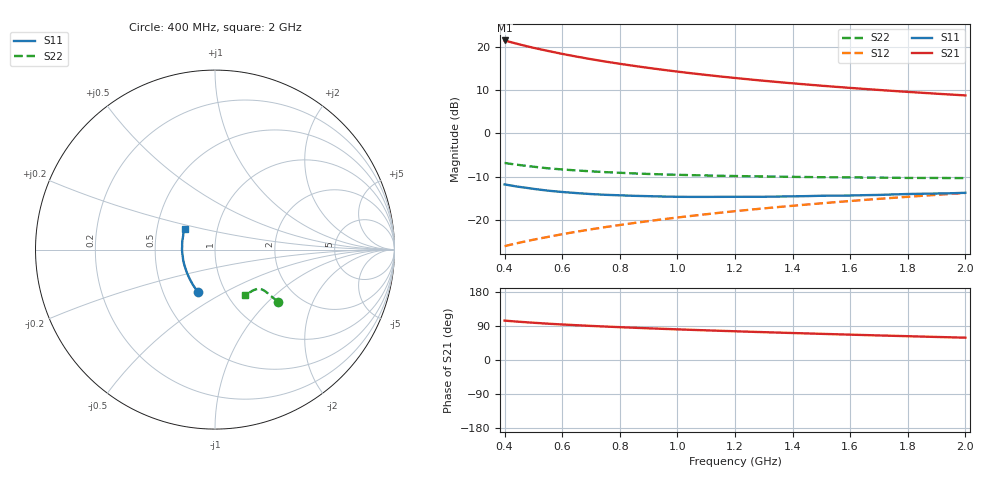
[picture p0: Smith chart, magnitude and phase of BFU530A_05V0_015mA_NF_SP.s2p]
! Filename:  P:\Prog\Test\Noise\ATS_data\Testdata_Net\06 Compressed Noise after Statistics\BFU530A_APG2013_33_A05_05p0V_015mA_NF_CM01_D.sf
! Date/Time: Tue 16/Apr/2013 15:10:56
! BFU530A_APG2013_33_A05_05p0V_1to25mA_NF_CM01_Bias6_R.sf
! Noise Parameter Data File
! BFU530A_APG2013_33_A05_05p0V_1to25mA_NF_CM01
! Date/time: Fri Apr 12 15:27:54 2013
! VAR V_out= 5.001000
! VAR I_out= 15.000000
! VAR V_in= 0.836900
! VAR I_in= 0.162200
! Device data file deembeded for feedlines and parallel
! Original file: \06 Compressed Noise after Statistics\BFU530A_APG2013_33_A05_05p0V_015mA_NF_CM01_R.sf
! Feed-files: PR017V01_150413_Feed1.s2p, PR017V01_150413_Feed2.s2p
! Parallel-file: PR017V01_150413_Par.s2p
# MHz S MA R 50
!  Freq-MHz  S11-mag  S11-arg  S21-mag  S21-arg  S12-mag  S12-arg  S22-mag  S22-arg
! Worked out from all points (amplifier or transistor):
!   37 points, 400 MHz to 2 GHz, reference 50 ohm
!   highest |S21| = 21.6 dB at 400 MHz (marker M1)
!   |S21| within 3 dB of that: start of sweep to 591.3 MHz
!   unconditionally stable (mu >= 1): 1.115 GHz to end of sweep
!   at 500 MHz: K = 0.89, MSG = 22.3 dB, |S12| = -24.7 dB
!   at 1.1 GHz: K = 1.00, MSG = 16.2 dB, |S12| = -18.8 dB
!   at 2 GHz: K = 1.00, MAG = 11.0 dB, |S12| = -13.8 dB
!   lowest NFmin = 0.91 dB at 460 MHz
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400  0.2556 -111.1  12.06 104.0  0.049 68.8  0.4546 -39.5
420  0.2493 -113.8  11.56 102.7  0.05089 69.0  0.4441 -39.6
440  0.2426 -116.7  11.11 101.5  0.05271 69.2  0.4349 -39.6
460  0.2374 -119.1  10.68 100.4  0.05455 69.4  0.4267 -39.7
500  0.2272 -124.2  9.917 98.3  0.05823 69.7  0.4112 -39.7
550  0.2167 -130.3  9.121 95.8  0.06276 70.0  0.3941 -39.6
600  0.2089 -135.3  8.421 93.7  0.0675 70.3  0.3821 -39.6
650  0.2029 -140.4  7.828 91.8  0.0722 70.6  0.3719 -39.7
700  0.1977 -144.8  7.311 90.0  0.07689 70.8  0.3631 -39.7
750  0.1937 -149.3  6.855 88.3  0.0816 70.9  0.3554 -39.8
800  0.1912 -153.3  6.458 86.7  0.08638 71.0  0.3494 -40.1
850  0.1885 -157.6  6.104 85.1  0.09113 71.0  0.3433 -40.4
900  0.1868 -161.3  5.785 83.6  0.09593 71.0  0.3384 -40.6
950  0.185 -164.8  5.5 82.2  0.1007 71.0  0.3347 -41.0
1050  0.1833 -171.4  5.005 79.5  0.1104 70.9  0.3278 -41.8
1150  0.1835 -177.5  4.597 77.0  0.1201 70.6  0.3222 -42.8
1200  0.1837 179.8  4.419 75.8  0.125 70.4  0.3203 -43.4
1350  0.185 172.0  3.96 72.3  0.1396 69.8  0.3151 -45.3
1500  0.1889 164.8  3.594 69.0  0.1543 69.0  0.3102 -47.4
1650  0.1919 158.7  3.294 65.8  0.1691 68.1  0.3077 -49.8
1750  0.1958 154.8  3.123 63.8  0.1788 67.5  0.3056 -51.5
2000  0.2044 146.2  2.771 58.9  0.2034 65.7  0.3031 -56.1
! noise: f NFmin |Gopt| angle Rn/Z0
400  0.9486  0.163  -168.2  0.0852
460  0.9082  0.171  -168  0.0848
600  0.9963  0.1595  -158.6  0.0985
800  0.9745  0.2248  -163.8  0.0746
1000  1.002  0.2207  -157.1  0.0801
1200  1.042  0.2242  -150.8  0.0857
1400  1.116  0.2504  -144.4  0.0785
1600  1.081  0.2691  -138.6  0.0904
1800  1.056  0.2899  -135.9  0.0947
2000  1.116  0.3138  -132.8  0.0924
